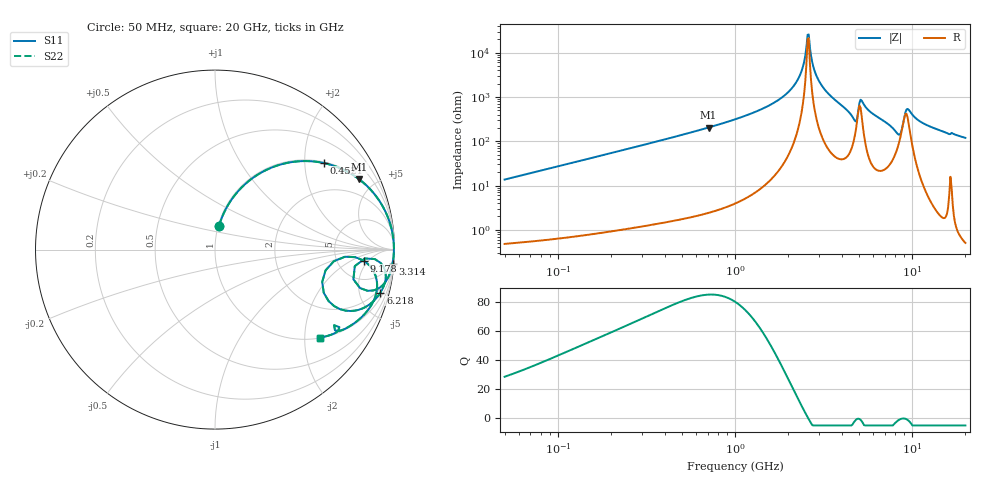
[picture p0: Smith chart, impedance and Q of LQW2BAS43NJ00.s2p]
!Murata Part Number: LQW2BAS43NJ00
!These Parameters are Measured in Series Mode Connection
!  o--[Z]--o
!Port1  Port2
!  o-------o
!Freq. Start=50[MHz] Stop=20[GHz], 401[Steps]
# Hz S RI R 50
!Freq.(Hz) S11(Real) S11(Imag) S21(Real) S21(Imag) S12(Real) S12(Imag) S22(Real) S22(Imag)
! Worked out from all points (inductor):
!   401 points, 50 MHz to 20 GHz, reference 50 ohm
!   read as one part in series: L = 43.2 nH near 51.52 MHz
!   highest Q = 84.8 at 708.6 MHz (marker M1), where L = 45.8 nH
!   self-resonance near 2.569 GHz
!   S11 on the Smith chart (normalised r, x): 50 MHz: 1.01, +0.27; 452.1 MHz: 1.03, +2.49; 3.314 GHz: 2, -25; 6.218 GHz: 1.47, -7.54; 9.178 GHz: 9, -4; 20 GHz: 1.01, -2.38
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5e7  0.0227 0.1324  0.9773 -0.1324  0.9773 -0.1324  0.0227 0.1324
1.364002e8  0.1246 0.3204  0.8754 -0.3204  0.8754 -0.3204  0.1246 0.3204
3.721004e8  0.508 0.4932  0.492 -0.4932  0.492 -0.4932  0.508 0.4932
4.520922e8  0.6067 0.4821  0.3933 -0.4821  0.3933 -0.4821  0.6067 0.4821
7.08568e8  0.8032 0.3917  0.1968 -0.3917  0.1968 -0.3917  0.8032 0.3917
1e9  0.9038 0.2887  0.0962 -0.2887  0.0962 -0.2887  0.9038 0.2887
1.544007e9  0.9727 0.1539  0.0273 -0.1539  0.0273 -0.1539  0.9727 0.1539
2.021818e9  0.9917 0.0733  0.00831 -0.0733  0.00831 -0.0733  0.9917 0.0733
2.348516e9  0.9961 0.0291  0.00386 -0.0291  0.00386 -0.0291  0.9961 0.0291
2.569357e9  0.9968 0.00234  0.00317 -0.00234  0.00317 -0.00234  0.9968 0.00234
2.647493e9  0.9967 -0.00668  0.00329 0.00668  0.00329 0.00668  0.9967 -0.00668
2.728004e9  0.9964 -0.0158  0.00358 0.0158  0.00358 0.0158  0.9964 -0.0158
2.940159e9  0.9949 -0.0388  0.00514 0.0388  0.00514 0.0388  0.9949 -0.0388
3.314454e9  0.9895 -0.0775  0.0105 0.0775  0.0105 0.0775  0.9895 -0.0775
4.677679e9  0.8502 -0.2295  0.1498 0.2295  0.1498 0.2295  0.8502 -0.2295
5.194772e9  0.9399 -0.0972  0.0601 0.0972  0.0601 0.0972  0.9399 -0.0972
6.217679e9  0.9216 -0.2397  0.0784 0.2397  0.0784 0.2397  0.9216 -0.2397
7.442007e9  0.815 -0.3306  0.185 0.3306  0.185 0.3306  0.815 -0.3306
8.389408e9  0.606 -0.2406  0.394 0.2406  0.394 0.2406  0.606 -0.2406
9.178299e9  0.8285 -0.0613  0.1715 0.0613  0.1715 0.0613  0.8285 -0.0613
1.183995e10  0.8459 -0.3451  0.1541 0.3451  0.1541 0.3451  0.8459 -0.3451
2e10  0.5862 -0.4904  0.4138 0.4904  0.4138 0.4904  0.5862 -0.4904
